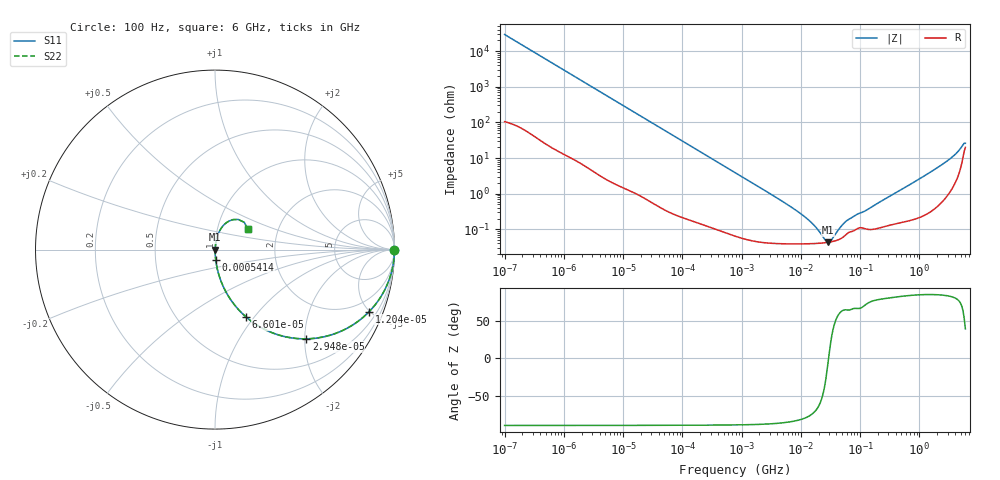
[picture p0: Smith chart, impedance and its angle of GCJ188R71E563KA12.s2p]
!Murata Part Number: GCJ188R71E563KA12
!These Parameters are Measured in Series Mode Connection
!Data Generated on Mar 13, 2026
!  o--ll--o
!Port1  Port2
!  o------o
!Operation Temp=25[degC], DC Bias Voltage=0[V]
!Freq. Start=100[Hz] Stop=6[GHz] 401[Steps]
# Hz S RI R 50
!Freq.(Hz) S11(Real) S11(Imag) S21(Real) S21(Imag) S12(Real) S12(Imag) S22(Real) S22(Imag)
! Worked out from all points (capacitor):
!   401 points, 100 Hz to 6 GHz, reference 50 ohm
!   read as one part in series: C = 53.9 nF near 109 Hz
!   lowest |Z| = 43.1 mohm at 29.12 MHz (marker M1)
!   series resonance near 29.41 MHz, so ESL is about 540 pH
!   S11 on the Smith chart (normalised r, x): 100 Hz: open; 12.04 kHz: 1.03, -4.96; 29.48 kHz: 1.01, -2.03; 66 kHz: 1.01, -0.91; 541.4 kHz: 1.00, -0.11; 6 GHz: 1.40, +0.33
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100  1 -0.00339  2.36e-05 0.00339  2.36e-05 0.00339  1 -0.00339
2008  0.9952 -0.0672  0.00484 0.0672  0.00484 0.0672  0.9952 -0.0672
6151  0.9584 -0.1974  0.0416 0.1974  0.0416 0.1974  0.9584 -0.1974
12041  0.8591 -0.3454  0.1409 0.3454  0.1409 0.3454  0.8591 -0.3454
18016  0.7329 -0.4397  0.2671 0.4397  0.2671 0.4397  0.7329 -0.4397
29482  0.5085 -0.4971  0.4915 0.4971  0.4915 0.4971  0.5085 -0.4971
40335  0.3572 -0.4763  0.6428 0.4763  0.6428 0.4763  0.3572 -0.4763
66005  0.1733 -0.3754  0.8267 0.3754  0.8267 0.3754  0.1733 -0.3754
141303  0.045 -0.2033  0.955 0.2033  0.955 0.2033  0.045 -0.2033
541393  0.00391 -0.0558  0.9961 0.0558  0.9961 0.0558  0.00391 -0.0558
774597  0.00218 -0.0391  0.9978 0.0391  0.9978 0.0391  0.00218 -0.0391
6644369  0.000408 -0.00436  0.9996 0.00436  0.9996 0.00436  0.000408 -0.00436
1.555665e7  0.000397 -0.00142  0.9996 0.00142  0.9996 0.00142  0.000397 -0.00142
2.545746e7  0.000418 -0.000302  0.9996 0.000302  0.9996 0.000302  0.000418 -0.000302
2.911731e7  0.000431 -2.05e-05  0.9996 2.05e-05  0.9996 2.05e-05  0.000431 -2.05e-05
3.330331e7  0.000448 0.000262  0.9996 -0.000262  0.9996 -0.000262  0.000448 0.000262
4.556224e7  0.00053 0.000956  0.9995 -0.000956  0.9995 -0.000956  0.00053 0.000956
5.960426e7  0.000741 0.00158  0.9993 -0.00158  0.9993 -0.00158  0.000741 0.00158
3.124326e8  0.00136 0.00825  0.9986 -0.00825  0.9986 -0.00825  0.00136 0.00825
3.352442e9  0.0204 0.0936  0.9796 -0.0936  0.9796 -0.0936  0.0204 0.0936
4.586474e9  0.0535 0.1414  0.9465 -0.1414  0.9465 -0.1414  0.0535 0.1414
6e9  0.1823 0.1129  0.8177 -0.1129  0.8177 -0.1129  0.1823 0.1129
